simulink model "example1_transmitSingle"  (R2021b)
settings: Solver=FixedStepDiscrete  StartTime=0.0  StopTime=inf  FixedStep=0.2  RelTol=1e-3
undefined symbols (not defined in the file or in its folder): Endian, Little
libraries: CANBusLib x4

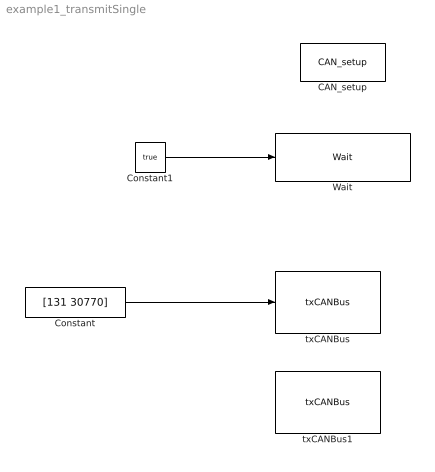
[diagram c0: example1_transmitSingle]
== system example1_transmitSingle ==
  CAN_setup : CANBusLib/CAN_setup  Priority=1  g1_cmbPortName="\"COM17\""  g2_cmbBaudRate=250000  g3_chkEcho=off  g59_chkTerminator=on  g4_cmbObjectID=0  g5_chkEnableSync=off  g10_chkRxWDEnable=off  g12_cmbRxWDLen=1  g13_cmbRxWDStartPos=1  g_60_cmbRxWDMode=0  g15_chkTxWDEnable=off  g17_cmbTxWDLen=1  g18_cmbTxWDStartPos=1  g_61_cmbTxWDMode=0  g20_ediF1=0  g21_chkExt4F1=off  g22_ediF2=0  g23_chkExt4F2=off  g24_ediF3=0  g25_chkExt4F3=off  g26_ediF4=0  g27_chkExt4F4=off  g28_ediF5=0  g29_chkExt4F5=off  g30_ediF6=0  g31_chkExt4F6=off  g32_ediF7=0  g33_chkExt4F7=off  g34_ediF8=0  g35_chkExt4F8=off  g36_ediM1=0  g37_ediF9=0  g38_chkExt4F9=on  g39_ediF10=0  g40_chkExt4F10=on  g41_ediF11=0  g42_chkExt4F11=on  g43_ediF12=0  g44_chkExt4F12=on  g45_ediM2=0  g46_ediF13=0  g47_chkExt4F13=off  g48_ediF14=0  g49_chkExt4F14=on  g50_ediF15=0  g51_chkExt4F15=on  g52_ediF16=0  g53_chkExt4F16=on  g54_ediM3=0  g62_autoFresh=on
  Constant : Constant  Value=[131 30770]
  Constant1 : Constant  Value=true
  Wait : CANBusLib/Wait  Waitms=200
  txCANBus : CANBusLib/txCANBus  g1_cmbObjectID=0  g2_CANID=68  g3_Extended=off  g4_RTR=off  g5_Datatype="[\"uint8\", \"uint16\"]"  g6_Endian=Little-Endian  g7_Longframe=off  g8_FirstFrameNo=1  g9_LastFrameDLC8=on
  txCANBus1 : CANBusLib/txCANBus  g1_cmbObjectID=0  g2_CANID=86  g3_Extended=on  g4_RTR=on  g5_Datatype="[\"uint8\", \"uint16\"]"  g6_Endian=Little-Endian  g7_Longframe=off  g8_FirstFrameNo=1  g9_LastFrameDLC8=on
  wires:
  Constant1/1 -> Wait/1
  Constant/1 -> txCANBus/1
